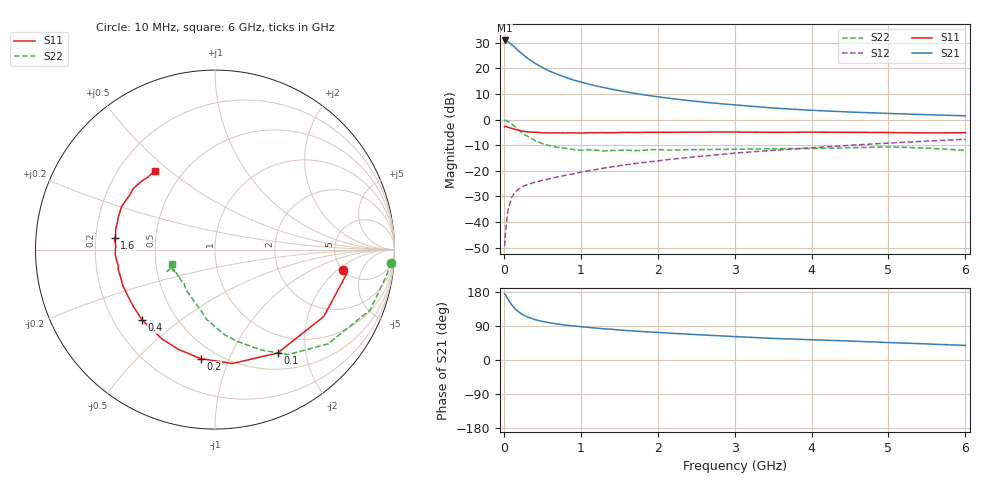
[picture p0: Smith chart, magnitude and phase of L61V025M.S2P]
!  INFINEON TECHNOLOGIES Small Signal Semiconductors
! BFR380L3 , Si-NPN RF-Transistor in TSLP-3-1
!  Vce=1 V,  Ic=25 mA
! Common Emitter S-Parameters:  07. March 2005
#  GHz  S  MA  R  50
! f  S11  S21  S12  S22
! GHz  Mag  Ang  Mag  Ang  Mag  Ang  Mag  Ang
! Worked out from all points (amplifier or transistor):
!   36 points, 10 MHz to 6 GHz, reference 50 ohm
!   highest |S21| = 30.8 dB at 10 MHz (marker M1)
!   |S21| within 3 dB of that: start of sweep to 154.6 MHz
!   unconditionally stable (mu >= 1): 1.681 GHz to 5.244 GHz
!   at 250 MHz: K = 0.40, MSG = 25.7 dB, |S12| = -26.0 dB
!   at 1.4 GHz: K = 0.97, MSG = 15.2 dB, |S12| = -18.5 dB
!   at 6 GHz: K = 0.99, MSG = 4.6 dB, |S12| = -7.7 dB
!   S11 on the Smith chart (normalised r, x): 10 MHz: 5.02, -2.36; 100 MHz: 0.72, -1.52; 200 MHz: 0.41, -0.79; 400 MHz: 0.32, -0.37; 1.6 GHz: 0.28, +0.05; 6 GHz: 0.35, +0.45
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0.01  0.7208 -9.0  34.84 174.4  0.0034 84.9  0.9842 -4.3
0.02  0.7462 -10.3  34.77 172.7  0.0059 84.5  0.9653 -8.8
0.05  0.7117 -31.6  33.13 161.6  0.0161 78.2  0.9274 -21.3
0.1  0.6735 -58.8  29.17 146.3  0.03 65.7  0.8197 -39.9
0.15  0.642 -81.2  25.03 134.3  0.039 57.2  0.7126 -55.2
0.2  0.6127 -97.5  21.32 125.7  0.0449 53.0  0.6139 -65.5
0.25  0.5918 -110.4  18.41 119.3  0.0499 49.9  0.5304 -75.7
0.3  0.5786 -120.7  15.98 114.2  0.0536 49.2  0.4802 -83.3
0.4  0.565 -135.8  12.62 106.8  0.0595 48.6  0.3925 -96.7
0.5  0.5541 -145.8  10.37 101.9  0.0652 49.6  0.3387 -104.8
0.6  0.5498 -153.2  8.718 97.9  0.0702 50.9  0.3094 -112.4
0.7  0.5512 -158.6  7.572 94.9  0.0763 52.5  0.2877 -119.6
0.9  0.5504 -168.3  5.944 89.9  0.0871 55.2  0.2611 -130.8
1.1  0.5525 -174.0  4.924 85.9  0.1006 57.5  0.2573 -136.3
1.3  0.5558 -179.9  4.206 82.3  0.1131 58.9  0.2445 -143.8
1.6  0.5629 173.6  3.437 77.7  0.1322 60.1  0.2517 -149.9
2.2  0.5648 164.2  2.546 70.3  0.1698 61.6  0.2539 -152.6
2.8  0.5734 155.5  2.048 63.9  0.2074 62.0  0.2616 -157.5
3.5  0.5639 147.1  1.679 57.0  0.2507 60.3  0.2702 -156.7
4.5  0.564 140.7  1.403 50.0  0.3152 58.6  0.2817 -156.2
5.5  0.5492 132.6  1.243 42.4  0.3801 54.8  0.2775 -156.9
6  0.554 127.3  1.184 38.5  0.4126 52.5  0.2513 -161.0
